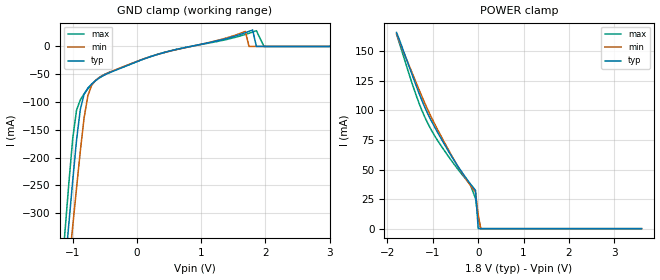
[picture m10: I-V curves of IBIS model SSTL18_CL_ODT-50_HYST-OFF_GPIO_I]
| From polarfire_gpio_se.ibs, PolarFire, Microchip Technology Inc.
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|   Model SSTL18_CL_ODT-50_HYST-OFF_GPIO_I
[Model]   SSTL18_CL_ODT-50_HYST-OFF_GPIO_I
Model_type   Input
Vinl =   0.775
Vinh =   1.025
|   typ   min   max
C_comp_pullup   2.605e-12   2.605e-12   2.76e-12
C_comp_pulldown  2.605e-12   2.605e-12   2.76e-12
[Temperature Range]  25C   100C   -40C
[Voltage Range]  1.8   1.71   1.89
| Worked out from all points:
|   POWER clamp passes 1 mA (typ) near -0.00 V on its own axis
[GND Clamp]
| Voltage   I(typ)   I(min)   I(max)
-1.8V     -1.272A    -1.24A     -1.324A
-1.122V   -393.6mA   -459.4mA   -329.1mA
-1.063V   -317.2mA   -391.4mA   -244.2mA
-1.004V   -241.2mA   -323.4mA   -165.6mA
-885.9mV  -113.4mA   -188.3mA   -95.96mA
-767.8mV  -74.77mA   -88.51mA   -76.15mA
-531.6mV  -52.72mA   -51.99mA   -51.66mA
1.688V    24.74mA    26.97mA    21.65mA
1.8V      29.61mA    0A         25.91mA
1.859V    0A         0A         28.31mA
1.977V    0A         0A         0A
3.6V      0A         0A         0A
[POWER Clamp]
| Voltage   I(typ)   I(min)   I(max)
-1.8V     166mA      164.9mA    164.5mA
-1.417V   126.1mA    128.2mA    118.3mA
-1.24V    108.3mA    111.8mA    99.92mA
-1.122V   98.04mA    101.4mA    89.93mA
-945mV    84.87mA    87.49mA    77.6mA
-649.7mV  65.09mA    66.25mA    60.76mA
-413.4mV  50.78mA    50.52mA    48.58mA
-177.2mV  38.13mA    36.88mA    37.45mA
-59.06mV  32.36mA    30.82mA    25.45mA
0V        0A         11.84mA    8.749mA
56.25mV   0A         0A         0A
3.6V      0A         0A         0A
